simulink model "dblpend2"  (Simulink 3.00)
settings: Solver=ode45  SolverMode=SingleTasking  StartTime=0  StopTime=10000  MaxStep=0.05  RelTol=1e-5  AbsTol=1e-6
PreLoadFcn:
  | l2=58.4154;w2=14.5619;n=1.084;e=.1478;

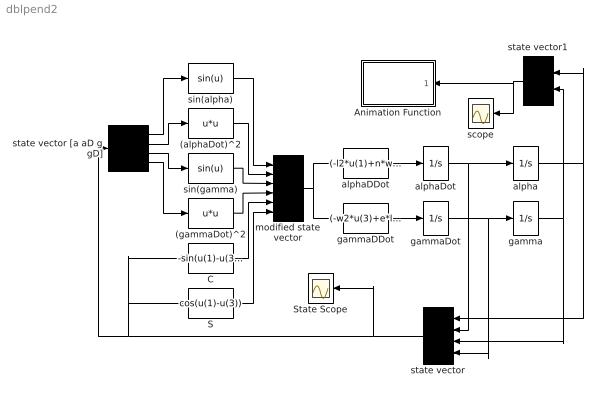
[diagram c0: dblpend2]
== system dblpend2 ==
  (alphaDot)^2 : Fcn  Expr=u*u
  (gammaDot)^2 : Fcn  Expr=u*u
  Animation Function : Subsystem  Orientation=left
  C : Fcn  Expr=-sin(u(1)-u(3))
  S : Fcn  Expr=cos(u(1)-u(3))
  State Scope : Scope
  alpha : Integrator  ExternalReset=none  InitialConditionSource=internal  InitialCondition=0*(pi/180)  LimitOutput=off  UpperSaturationLimit=inf  LowerSaturationLimit=-inf  ShowSaturationPort=off  ShowStatePort=off  AbsoluteTolerance=auto
  alphaDDot : Fcn  Expr=(-l2*u(1)+n*w2*u(5)*u(3)-n*e*u(5)*u(6)*u(2)-n*u(6)*u(4))/(1-n*e*u(5)*u(5))
  alphaDot : Integrator  ExternalReset=none  InitialConditionSource=internal  InitialCondition=0  LimitOutput=off  UpperSaturationLimit=inf  LowerSaturationLimit=-inf  ShowSaturationPort=off  ShowStatePort=off  AbsoluteTolerance=auto
  gamma : Integrator  ExternalReset=none  InitialConditionSource=internal  InitialCondition=80*(pi/180)  LimitOutput=off  UpperSaturationLimit=inf  LowerSaturationLimit=-inf  ShowSaturationPort=off  ShowStatePort=off  AbsoluteTolerance=auto
  gammaDDot : Fcn  Expr=(-w2*u(3)+e*l2*u(5)*u(1)+n*e*u(5)*u(6)*u(4)+e*u(6)*u(2))/(1-n*e*u(5)*u(5))
  gammaDot : Integrator  ExternalReset=none  InitialConditionSource=internal  InitialCondition=0  LimitOutput=off  UpperSaturationLimit=inf  LowerSaturationLimit=-inf  ShowSaturationPort=off  ShowStatePort=off  AbsoluteTolerance=auto
  modified state vector : Mux  Inputs=6
  scope : Scope
  sin(alpha) : Fcn  Expr=sin(u)
  sin(gamma) : Fcn  Expr=sin(u)
  state vector : Mux  Orientation=left  Inputs=4
  state vector [a aD g gD] : Demux  Outputs=4
  state vector1 : Mux  Orientation=left  Inputs=2
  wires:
  alphaDDot/1 -> alphaDot/1
  gammaDDot/1 -> gammaDot/1
  alphaDot/1 -> alpha/1, state vector/2
  gammaDot/1 -> gamma/1, state vector/4
  alpha/1 -> state vector/1, state vector1/1
  gamma/1 -> state vector/3, state vector1/2
  state vector1/1 -> Animation Function/1(In1), scope/1
  state vector/1 -> state vector [a aD g gD]/1, C/1, S/1, State Scope/1
  sin(alpha)/1 -> modified state vector/1
  (alphaDot)^2/1 -> modified state vector/2
  sin(gamma)/1 -> modified state vector/3
  (gammaDot)^2/1 -> modified state vector/4
  C/1 -> modified state vector/5
  S/1 -> modified state vector/6
  modified state vector/1 -> alphaDDot/1, gammaDDot/1
  state vector [a aD g gD]/4 -> (gammaDot)^2/1
  state vector [a aD g gD]/3 -> sin(gamma)/1
  state vector [a aD g gD]/2 -> (alphaDot)^2/1
  state vector [a aD g gD]/1 -> sin(alpha)/1

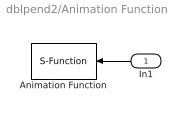
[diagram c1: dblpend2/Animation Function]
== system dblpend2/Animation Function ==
  In1 : Inport  Orientation=left  Port=1  PortWidth=-1  SampleTime=-1  DataType=auto
  Animation Function : S-Function  Orientation=left  FunctionName=pndanim3  Parameters=0.05  PortCounts=[]  SFunctionModules=''
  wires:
  In1/1 -> Animation Function/1
